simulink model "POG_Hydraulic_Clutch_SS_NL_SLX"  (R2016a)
settings: Solver=ode45  StartTime=0.0  StopTime=10.0  MaxStep=0.001  RelTol=1e-3
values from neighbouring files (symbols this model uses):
  A = 5*cm^2    (= 0.0005)    [POG_Hydraulic_Clutch_NL_2_SLX_m.m]    (also in POG_Hydraulic_Clutch_SS_NL_SLX_m.m = 5*cm^2; POG_Hydraulic_Clutch_SS_SLX_m.m = 1)
  b_p = 10    [POG_Hydraulic_Clutch_NL_2_SLX_m.m]    (also in POG_Hydraulic_Clutch_SS_NL_SLX_m.m; POG_Hydraulic_Clutch_SS_SLX_m.m = 1)
  C_m = 1e-9    (= 1e-09)    [POG_Hydraulic_Clutch_NL_2_SLX_m.m]    (also in POG_Hydraulic_Clutch_SS_NL_SLX_m.m; POG_Hydraulic_Clutch_SS_SLX_m.m = 1; POG_Hydraulic_Clutch_SS_When_Cm_is_0.m = 0)
  K_m = P_a_t*A/(3*cm)    (= 16887.5)    [POG_Hydraulic_Clutch_NL_2_SLX_m.m]    (also in POG_Hydraulic_Clutch_SS_NL_SLX_m.m = P_a_0*A/(3*cm); POG_Hydraulic_Clutch_SS_SLX_m.m = 1; POG_Electro_Hydraulic_Pump_NL_SLX_m.m = 0.5; POG_Electro_Hydraulic_Pump_Rele_SLX_m.m = 0.5)
  K_v = (80*cm)^3/(sec*(0.2*atm))    (= 2.52652356279e-05)    [POG_Hydraulic_Clutch_NL_2_SLX_m.m]    (also in POG_Hydraulic_Clutch_SS_NL_SLX_m.m = (10*cm)^3/(sec*(0.2*atm)); POG_Hydraulic_Clutch_SS_SLX_m.m = 1)
  m_p = 300*gr    (= 0.3)    [POG_Hydraulic_Clutch_NL_2_SLX_m.m]    (also in POG_Hydraulic_Clutch_SS_NL_SLX_m.m = 300*gr; POG_Hydraulic_Clutch_SS_SLX_m.m = 1)
  P_6_0 = 0    [POG_Hydraulic_Clutch_SS_NL_SLX_m.m]    (also in POG_Hydraulic_Clutch_SS_SLX_m.m; POG_Electro_Hydraulic_Pump_NL_SLX_m.m; POG_Electro_Hydraulic_Pump_Rele_SLX_m.m; POG_Electro_Hydraulic_Pump_SLX_m.m)
  P_a_0 = 10*atm    [POG_Hydraulic_Clutch_SS_NL_SLX_m.m]    (also in POG_Hydraulic_Clutch_SS_SLX_m.m = 1000)
  Ts = Tfin/Nr_Ts_Points    (= 0.0002)    [POG_Hydraulic_Clutch_NL_2_SLX_m.m]    (also in POG_Hydraulic_Clutch_SS_NL_SLX_m.m; POG_Hydraulic_Clutch_SS_SLX_m.m = 0.005; POG_Electro_Hydraulic_Pump_NL_SLX_m.m = 0.03; POG_Electro_Hydraulic_Pump_Rele_SLX_m.m = 0.035)
  V_3_0 = 0    [POG_Hydraulic_Clutch_SS_NL_SLX_m.m]    (also in POG_Hydraulic_Clutch_SS_SLX_m.m)
  v_d_0 = 0    [POG_Hydraulic_Clutch_SS_NL_SLX_m.m]    (also in POG_Hydraulic_Clutch_SS_SLX_m.m)
  x_8_0 = 0    [POG_Hydraulic_Clutch_SS_NL_SLX_m.m]    (also in POG_Hydraulic_Clutch_SS_SLX_m.m)

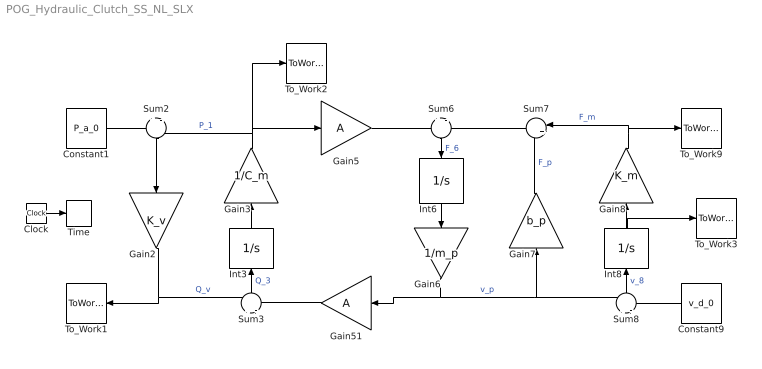
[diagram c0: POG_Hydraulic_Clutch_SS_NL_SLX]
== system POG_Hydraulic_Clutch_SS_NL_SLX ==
  Clock : Clock
  Constant1 : Constant  Value=P_a_0
  Constant9 : Constant  Value=v_d_0
  Gain2 : Gain  Gain=K_v  Multiplication=Matrix(K*u)
  Gain3 : Gain  Gain=1/C_m  Multiplication=Matrix(K*u)
  Gain5 : Gain  Gain=A  Multiplication=Matrix(K*u)
  Gain51 : Gain  Gain=A  Multiplication=Matrix(K*u)
  Gain6 : Gain  Gain=1/m_p  Multiplication=Matrix(K*u)
  Gain7 : Gain  Gain=b_p  Multiplication=Matrix(K*u)
  Gain8 : Gain  Gain=K_m  Multiplication=Matrix(K*u)
  Int3 : Integrator  InitialCondition=V_3_0
  Int6 : Integrator  InitialCondition=P_6_0
  Int8 : Integrator  InitialCondition=x_8_0
  Sum{2..3,6,8} (4 alike) : Sum  Inputs=+|-
  Sum7 : Sum  Inputs=|++
  Time : ToWorkspace  VariableName=t  SampleTime=Ts
  To_Work1 : ToWorkspace  VariableName=Q_a_0  SampleTime=Ts
  To_Work2 : ToWorkspace  VariableName=P_1  SampleTime=Ts
  To_Work3 : ToWorkspace  VariableName=x_p  SampleTime=Ts
  To_Work9 : ToWorkspace  VariableName=F_d_0  SampleTime=Ts
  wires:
  Constant1/1 -> Sum2/1
  Gain3/1 -> To_Work2/1, Sum2/2, Gain5/1  "P_1"
  Gain2/1 -> To_Work1/1, Sum3/1  "Q_v"
  Sum2/1 -> Gain2/1
  Gain51/1 -> Sum3/2
  Sum3/1 -> Int3/1  "Q_3"
  Int3/1 -> Gain3/1
  Gain5/1 -> Sum6/1
  Gain6/1 -> Gain51/1, Gain7/1, Sum8/1  "v_p"
  Sum7/1 -> Sum6/2
  Sum6/1 -> Int6/1  "F_6"
  Int6/1 -> Gain6/1
  Gain8/1 -> Sum7/1, To_Work9/1  "F_m"
  Gain7/1 -> Sum7/2  "F_p"
  Constant9/1 -> Sum8/2
  Sum8/1 -> Int8/1  "v_8"
  Int8/1 -> To_Work3/1, Gain8/1
  Clock/1 -> Time/1
